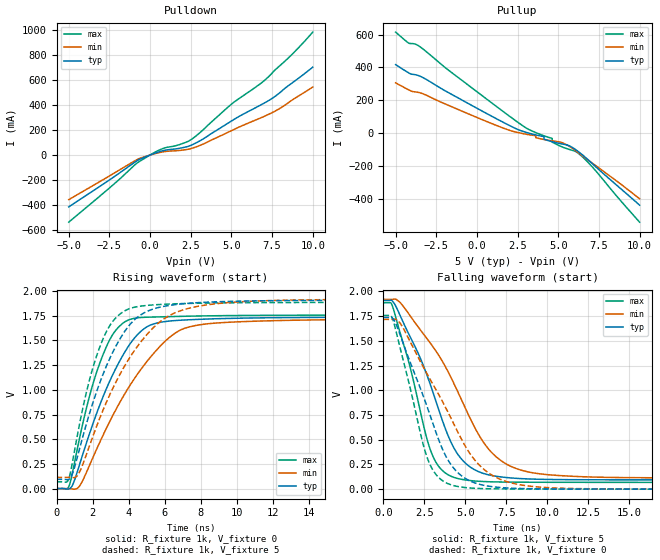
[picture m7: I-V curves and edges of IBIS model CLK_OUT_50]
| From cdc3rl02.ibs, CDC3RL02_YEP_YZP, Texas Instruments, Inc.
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[Model]   CLK_OUT_50
Model_type  Output
Vref =   1.8
Rref =   1M
Cref =   30p
Vmeas =   0.9
| variable   typ   min   max
C_comp   37.81pF   28.62pF   49.62pF
| C_pullup   34.06pF   28.62pF   37.29pF
| C_pulldown   41.57pF   34.13pF   49.62pF
[Temperature Range]   40   100   -40
| Ambient temperature   25   85   -40
[Voltage range]   5   4.5   5.5
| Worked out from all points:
|   slope of the pulldown table from 0 to 0.75 V, typ, clamps not added: 22.5 ohm
|   slope of the pullup table from 0 to 0.75 V, typ, clamps not added: 18.7 ohm
|   rising waveform, R_fixture 1k, V_fixture 0: 20-80 % time 2.35ns typ, 3.32ns min, 1.6ns max; typ from 0 V to 1.74 V
|   falling waveform, R_fixture 1k, V_fixture 5: 20-80 % time 2.56ns typ, 3.61ns min, 1.67ns max; typ from 1.91 V to 0.094 V
|   rising waveform, R_fixture 1k, V_fixture 5: 20-80 % time 2.26ns typ, 3.1ns min, 1.55ns max; typ from 0.094 V to 1.91 V
|   falling waveform, R_fixture 1k, V_fixture 0: 20-80 % time 2.37ns typ, 3.35ns min, 1.55ns max; typ from 1.74 V to 0 V
[Pulldown]
| CLK_OUT_50
|   Voltage   I(typ)   I(min)   I(max)
-5V       -414mA     -356.5mA   -536.5mA
-2.345V   -185.4mA   -155.2mA   -246.3mA
-745mV    -41.18mA   -32.75mA   -59.49mA
580mV     27.21mA    19.99mA    40.83mA
2.105V    61.71mA    41.3mA     97.08mA
2.405V    72.27mA    48.02mA    113.9mA
2.775V    93.59mA    62.61mA    147.5mA
5.02V     273.4mA    195.9mA    408.3mA
7.11V     421.7mA    314.5mA    604.8mA
7.94V     494.5mA    369.4mA    709.4mA
8.785V    581mA      443.9mA    811.9mA
10V       701.9mA    543.3mA    982.4mA
[Pullup]
| CLK_OUT_50
|   Voltage   I(typ)   I(min)   I(max)
-5V       417.6mA    306.5mA    615.4mA
-4.195V   367.1mA    264mA      548.5mA
-3.435V   344mA      243.9mA    521.4mA
1.15V     90.38mA    48.9mA     166.3mA
2.875V    9.525mA    -3.559mA   41.31mA
4.12V     -20.86mA   -38.72mA   -16.15mA
4.125V    -36.77mA   -38.81mA   -16.32mA
4.625V    -52.34mA   -46.64mA   -31.67mA
4.63V     -52.48mA   -46.71mA   -55.31mA
5.22V     -65.58mA   -57.24mA   -82.98mA
6.24V     -112.9mA   -119.3mA   -123.7mA
10V       -438.5mA   -399.7mA   -542mA
[Ramp]
| CLK_OUT_50
| variable   typ   min   max
dV/dt_r   1.05/2.36E-09   1.03/3.33E-09   1.06/1.60E-09
dV/dt_f   1.09/2.57E-09   1.09/3.62E-09   1.09/1.67E-09
R_load = 1k
[Rising Waveform]
| CLK_OUT_50
R_fixture =   1k
C_fixture =   0
L_fixture =   0
V_fixture =   0
V_fixture_min = 0
V_fixture_max = 0
|   Time   V(typ)   V(min)   V(max)
0s        9.559nV    28.61nV    2.329nV
709ps     -2.007mV   -228.2uV   32.54mV
1.301ns   256.5mV    31.81mV    530.2mV
2.029ns   661.9mV    319.1mV    1.065V
2.797ns   1.025V     622.4mV    1.449V
4.221ns   1.501V     1.087V     1.721V
5.109ns   1.648V     1.309V     1.736V
6.397ns   1.699V     1.55V      1.742V
8.413ns   1.717V     1.67V      1.749V
37.7ns    1.737V     1.717V     1.757V
[Falling Waveform]
| CLK_OUT_50
R_fixture =   1k
C_fixture =   0
L_fixture =   0
V_fixture =   5
V_fixture_min = 4.5
V_fixture_max = 5.5
|   Time   V(typ)   V(min)   V(max)
0s        1.909V     1.92V      1.886V
581ps     1.896V     1.92V      1.838V
1.053ns   1.745V     1.882V     1.563V
2.973ns   1.004V     1.452V     351mV
3.525ns   730.6mV    1.314V     201mV
4.469ns   370.5mV    1.01V      110.8mV
5.349ns   218.1mV    697.5mV    86.14mV
6.549ns   140.1mV    380.5mV    74.57mV
9.197ns   101.4mV    163.2mV    69.88mV
37.7ns    93.62mV    113.4mV    68.51mV
[Rising Waveform]
| CLK_OUT_50
R_fixture =   1k
C_fixture =   0
L_fixture =   0
V_fixture =   5
V_fixture_min = 4.5
V_fixture_max = 5.5
|   Time   V(typ)   V(min)   V(max)
0s        93.63mV    113.4mV    68.52mV
701ps     95.76mV    113.2mV    111.7mV
1.309ns   424.4mV    179.7mV    683.1mV
1.949ns   830.7mV    494.4mV    1.181V
2.597ns   1.165V     802.3mV    1.523V
3.301ns   1.445V     1.081V     1.731V
4.253ns   1.697V     1.38V      1.834V
6.253ns   1.855V     1.751V     1.869V
9.261ns   1.894V     1.879V     1.881V
37.7ns    1.908V     1.919V     1.886V
[Falling Waveform]
| CLK_OUT_50
R_fixture =   1k
C_fixture =   0
L_fixture =   0
V_fixture =   0
V_fixture_min = 0
V_fixture_max = 0
|   Time   V(typ)   V(min)   V(max)
0s        1.737V     1.717V     1.757V
621ps     1.716V     1.719V     1.692V
1.173ns   1.49V      1.64V      1.327V
2.765ns   787.4mV    1.136V     278.8mV
3.573ns   416.9mV    896.1mV    89.88mV
4.277ns   215.1mV    666.6mV    36.51mV
5.237ns   86.8mV     370.5mV    12.55mV
6.149ns   38.34mV    198.1mV    5.494mV
8.861ns   4.932mV    31.87mV    1.323mV
37.7ns    -9.786uV   -13.07uV   -6.671uV
